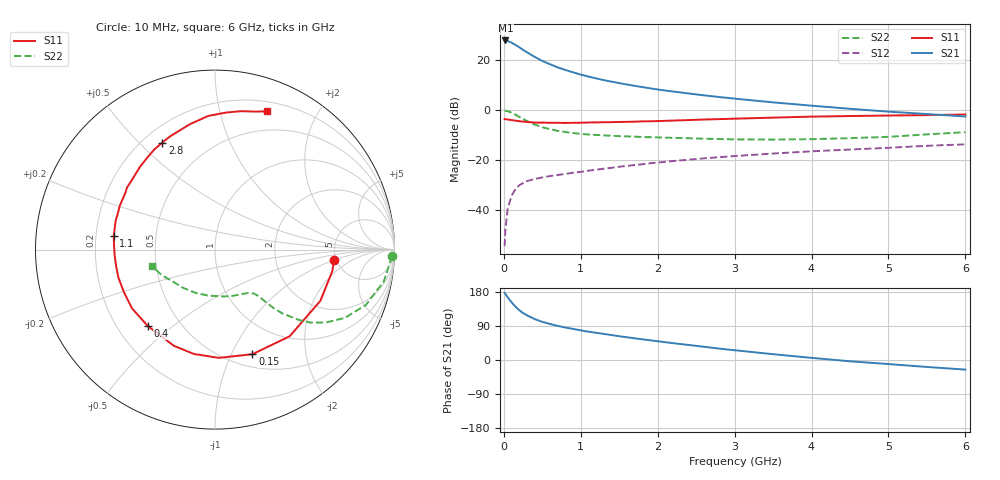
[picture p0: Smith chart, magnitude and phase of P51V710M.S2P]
! SIEMENS Small Signal Semiconductors
! BFP183
! Si NPN RF Bipolar Junction Transistor in SOT143
! VCE = 1.75 V  IC = 10 mA
! Common Emitter S-Parameters:  March  1996
# GHz  S  MA  R  50
!  f  S11  S21  S12  S22
! GHz  MAG  ANG  MAG  ANG  MAG  ANG  MAG  ANG
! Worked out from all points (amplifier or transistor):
!   36 points, 10 MHz to 6 GHz, reference 50 ohm
!   highest |S21| = 28.0 dB at 20 MHz (marker M1)
!   |S21| within 3 dB of that: start of sweep to 213 MHz
!   unconditionally stable (mu >= 1): 1.117 GHz to 5.7 GHz
!   at 250 MHz: K = 0.33, MSG = 26.7 dB, |S12| = -29.2 dB
!   at 1.4 GHz: K = 1.10, MAG = 15.4 dB, |S12| = -23.0 dB
!   at 6 GHz: K = 0.96, MSG = 5.6 dB, |S12| = -13.7 dB
!   S11 on the Smith chart (normalised r, x): 10 MHz: 4.76, -1.01; 150 MHz: 0.64, -1.21; 400 MHz: 0.33, -0.41; 1.1 GHz: 0.28, +0.06; 2.8 GHz: 0.27, +0.59; 6 GHz: 0.29, +1.41
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0.01  0.6656 -5.1  24.86 177.2  0.0019 82.1  0.9846 -2.1
0.02  0.6648 -10.3  25 174.6  0.004 87.7  0.9772 -4.3
0.05  0.6527 -25.9  24.5 165.4  0.0106 81.2  0.9572 -10.7
0.1  0.6374 -49.3  22.53 152.4  0.0194 68.0  0.8949 -20.2
0.15  0.619 -70.3  20.44 140.8  0.0261 60.6  0.817 -27.8
0.2  0.6036 -87.9  18.27 131.5  0.0315 54.2  0.7381 -33.4
0.25  0.5933 -101.4  16.16 123.9  0.0348 49.6  0.6695 -37.4
0.3  0.583 -113.1  14.51 118.0  0.0382 47.0  0.6087 -40.0
0.4  0.567 -131.3  11.75 108.0  0.042 43.0  0.5185 -43.4
0.5  0.5666 -144.7  9.717 100.7  0.0452 40.9  0.458 -45.0
0.6  0.56 -155.0  8.357 95.0  0.0482 40.3  0.4177 -45.8
0.7  0.5604 -163.6  7.215 90.0  0.0506 40.8  0.3875 -46.2
0.9  0.56 -176.8  5.75 82.0  0.056 41.2  0.3499 -47.2
1.1  0.5693 172.2  4.741 74.7  0.0617 42.0  0.3273 -48.5
1.3  0.5764 163.6  4.012 68.7  0.0675 42.7  0.3142 -50.5
1.6  0.5862 151.7  3.282 60.0  0.0769 43.1  0.3003 -54.2
2.2  0.6217 132.4  2.373 44.4  0.0961 42.1  0.2798 -65.0
2.8  0.665 116.2  1.842 30.1  0.115 38.8  0.2662 -78.9
3.5  0.7123 101.4  1.439 15.3  0.136 34.6  0.259 -98.2
4.5  0.7662 85.3  1.071 -3.4  0.1636 27.0  0.2765 -129.0
5.5  0.8001 74.0  0.84 -18.4  0.1944 20.1  0.3292 -154.4
6  0.823 69.3  0.751 -25.3  0.2077 15.7  0.3639 -165.6
